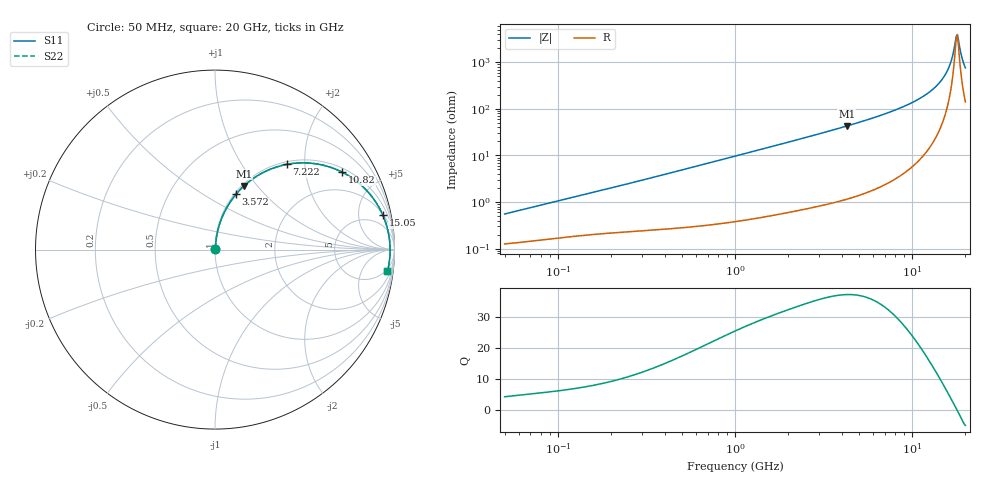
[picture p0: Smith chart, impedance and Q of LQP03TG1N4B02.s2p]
!Murata Part Number: LQP03TG1N4B02
!These Parameters are Measured in Series Mode Connection
!  o--[Z]--o
!Port1  Port2
!  o-------o
!Freq. Start=50[MHz] Stop=20[GHz], 401[Steps]
# Hz S RI R 50
!Freq.(Hz) S11(Real) S11(Imag) S21(Real) S21(Imag) S12(Real) S12(Imag) S22(Real) S22(Imag)
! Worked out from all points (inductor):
!   401 points, 50 MHz to 20 GHz, reference 50 ohm
!   read as one part in series: L = 1.69 nH near 51.52 MHz
!   highest Q = 37.3 at 4.276 GHz (marker M1), where L = 1.59 nH
!   self-resonance near 17.74 GHz
!   S11 on the Smith chart (normalised r, x): 50 MHz: 1.00, +0.01; 3.572 GHz: 1.02, +0.70; 7.222 GHz: 1.05, +1.62; 10.82 GHz: 1.15, +3.20; 15.05 GHz: 2.16, +9.40; 20 GHz: 4, -15
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5e7  0.00129 0.00537  0.9987 -0.00537  0.9987 -0.00537  0.00129 0.00537
1.364002e8  0.00209 0.0138  0.9979 -0.0138  0.9979 -0.0138  0.00209 0.0138
3.721004e8  0.00386 0.0361  0.9961 -0.0361  0.9961 -0.0361  0.00386 0.0361
1e9  0.0129 0.0948  0.9871 -0.0948  0.9871 -0.0948  0.0129 0.0948
2.728004e9  0.0717 0.2441  0.9283 -0.2441  0.9283 -0.2441  0.0717 0.2441
3.572216e9  0.1167 0.3078  0.8833 -0.3078  0.8833 -0.3078  0.1167 0.3078
4.275624e9  0.1615 0.3549  0.8385 -0.3549  0.8385 -0.3549  0.1615 0.3549
5.598765e9  0.2606 0.4254  0.7394 -0.4254  0.7394 -0.4254  0.2606 0.4254
7.222371e9  0.4002 0.4749  0.5998 -0.4749  0.5998 -0.4749  0.4002 0.4749
7.442007e9  0.4198 0.4782  0.5802 -0.4782  0.5802 -0.4782  0.4198 0.4782
9.041845e9  0.563 0.4779  0.437 -0.4779  0.437 -0.4779  0.563 0.4779
1.082228e10  0.7101 0.4308  0.2899 -0.4308  0.2899 -0.4308  0.7101 0.4308
1.314879e10  0.8596 0.3131  0.1404 -0.3131  0.1404 -0.3131  0.8596 0.3131
1.504638e10  0.9357 0.1911  0.0643 -0.1911  0.0643 -0.1911  0.9357 0.1911
1.621653e10  0.9621 0.1125  0.0379 -0.1125  0.0379 -0.1125  0.9621 0.1125
1.670968e10  0.9688 0.0796  0.0312 -0.0796  0.0312 -0.0796  0.9688 0.0796
1.747767e10  0.9747 0.0294  0.0253 -0.0294  0.0253 -0.0294  0.9747 0.0294
1.774144e10  0.9755 0.0125  0.0245 -0.0125  0.0245 -0.0125  0.9755 0.0125
1.800918e10  0.9758 -0.00439  0.0242 0.00439  0.0242 0.00439  0.9758 -0.00439
1.828096e10  0.9754 -0.0213  0.0246 0.0213  0.0246 0.0213  0.9754 -0.0213
1.940974e10  0.9681 -0.0883  0.0319 0.0883  0.0319 0.0883  0.9681 -0.0883
2e10  0.961 -0.1212  0.039 0.1212  0.039 0.1212  0.961 -0.1212
